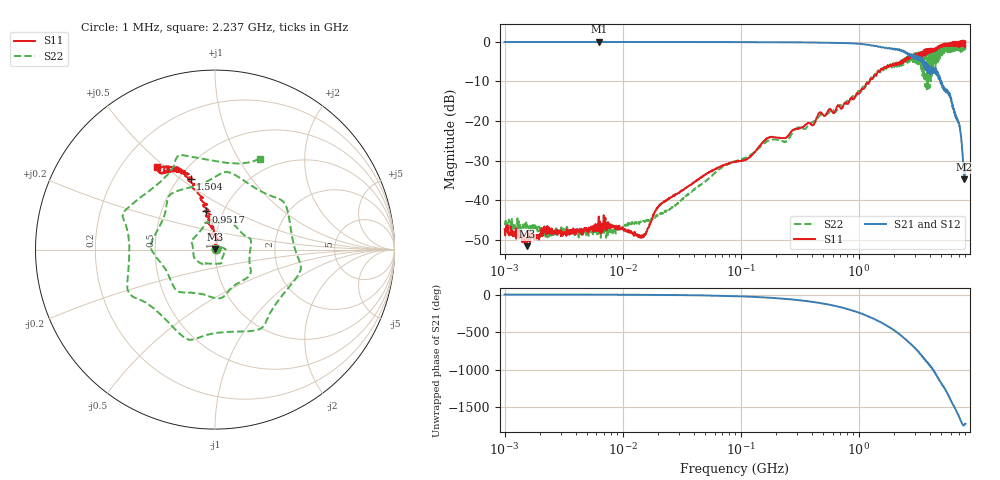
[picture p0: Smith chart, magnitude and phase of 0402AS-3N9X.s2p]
!s-Parameter Generated by FASTRON Sdn. Bhd.
!FASTRON P/N : 0402AS-3N9X
!Keysight Technologies: E5071C_MY46733604_B.14.02
!Date: Mon Dec 01 10:23:26 2025
!Version  :Rev00  Mon Dec 01 10:23:26 2025
!Data & Calibration Information:
!Freq  S11:SOLT2(ON)  S21:SOLT2(ON)  S12:SOLT2(ON)  S22:SOLT2(ON)
!PortZ  Port1:50+j0  Port2:50+j0
!When reading reference impedance value at option line is always used.
! Remarks : This data is being provided solely for informational purposes.
# Hz S dB R 50
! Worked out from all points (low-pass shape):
!   1601 points, 1 MHz to 8 GHz, reference 50 ohm
!   highest |S21| = 0.02 dB at 6.268 MHz (marker M1); lowest = -34.7 dB at 7.846 GHz (marker M2)
!   |S21| within 3 dB of the highest: start of sweep to 2.523 GHz; 2.541 GHz to 2.596 GHz (55.57 MHz wide, 2.16 % of centre)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
!   lowest |S11| = -51.6 dB at 1.541 MHz (marker M3), VSWR 1.01, Z = 50.2 + j0.116 ohm
!   |S11| at or under -10 dB: start of sweep to 1.231 GHz
!   |S22| runs from -49.5 to -0.6 dB; largest |S21 - S12| = 0.016
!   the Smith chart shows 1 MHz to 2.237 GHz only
!   S11 on the Smith chart (normalised r, x): 1 MHz: 1.01, +0.00; 951.7 MHz: 0.83, +0.37; 1.504 GHz: 0.57, +0.55; 2.237 GHz: 0.35, +0.47
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1000000  -47.30 24.2  -0.05 -0.3  -0.02 -0.3  -46.10 12.9
1541011  -51.60 26.0  -0.05 -0.4  -0.03 -0.4  -46.20 -4.5
4479405  -47.20 19.6  -0.05 -1.1  -0.03 -1.1  -48.00 23.1
6268472  -44.10 4.1  0.02 -1.6  -0.03 -2.1  -48.50 2.5
2.00676e7  -41.60 29.1  -0.05 -5.0  -0.05 -4.9  -43.60 54.6
8.994653e7  -30.30 88.7  -0.08 -21.9  -0.07 -21.9  -30.20 22.6
4.006501e8  -21.00 107.0  -0.18 -96.5  -0.17 -96.5  -20.40 -126.0
9.517328e8  -13.20 104.0  -0.45 131.0  -0.44 131.0  -13.80 -20.0
1.504228e9  -7.58 109.0  -1.23 -1.2  -1.22 -1.3  -7.63 66.4
1.7949e9  -6.40 114.0  -1.57 -69.1  -1.57 -69.2  -6.47 -74.1
2.007949e9  -5.88 122.0  -1.75 -120.0  -1.74 -120.0  -6.41 177.0
2.237469e9  -4.96 125.0  -2.24 -175.0  -2.22 -175.0  -4.95 63.8
2.545586e9  -4.26 128.0  -2.96 112.0  -2.93 112.0  -3.81 -84.4
2.750998e9  -3.93 130.0  -3.41 65.0  -3.37 64.9  -3.45 180.0
2.985754e9  -3.58 141.0  -3.68 7.2  -3.65 7.0  -5.15 49.6
3.26428e9  -3.81 145.0  -3.82 -59.5  -3.79 -59.7  -6.03 -74.7
3.487237e9  -2.41 151.0  -5.64 -114.0  -5.60 -115.0  -6.16 141.0
3.771001e9  -1.83 155.0  -7.49 -179.0  -7.45 -180.0  -12.00 10.1
4.216915e9  -2.58 162.0  -6.51 85.6  -6.52 85.0  -1.70 -174.0
4.548578e9  -1.48 162.0  -8.29 6.4  -8.35 6.0  -5.22 39.0
7.845781e9  -0.76 -76.8  -34.70 71.1  -34.70 71.5  -0.55 -126.0
8e9  0.08 -86.8  -30.80 81.0  -30.90 81.2  -1.90 160.0
